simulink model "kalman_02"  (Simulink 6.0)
settings: Solver=FixedStepDiscrete  StartTime=0.0  StopTime=499  FixedStep=1  RelTol=1e-3
libraries: simulink x1

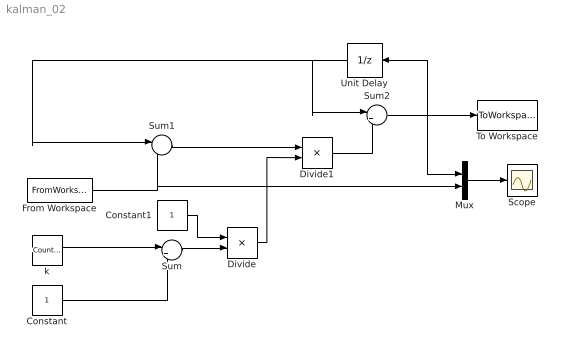
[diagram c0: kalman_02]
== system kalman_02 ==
  Constant : Constant
  Constant1 : Constant
  Divide : Product  Inputs=*/  OutScaling=2^-10
  Divide1 : Product  Inputs=**  OutScaling=2^-10
  From Workspace : FromWorkspace  VariableName=[t,z]  SampleTime=1
  Mux : Mux  Inputs=2
  Scope : Scope
  Sum : Sum  Inputs=|++
  Sum1 : Sum  Inputs=|-+
  Sum2 : Sum  Inputs=|++
  To Workspace : ToWorkspace  VariableName=simout  SampleTime=-1  SaveFormat=Array
  Unit Delay : UnitDelay  Orientation=left
  k : simulink/Sources/Counter Limited  uplimit=1000  tsamp=1
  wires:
  k/1 -> Sum/1
  Constant/1 -> Sum/2
  Sum/1 -> Divide/2
  Constant1/1 -> Divide/1
  Divide/1 -> Divide1/2
  From Workspace/1 -> Sum1/2, Mux/2
  Divide1/1 -> Sum2/2
  Sum2/1 -> Unit Delay/1, To Workspace/1, Mux/1
  Unit Delay/1 -> Sum2/1, Sum1/1
  Sum1/1 -> Divide1/1
  Mux/1 -> Scope/1
